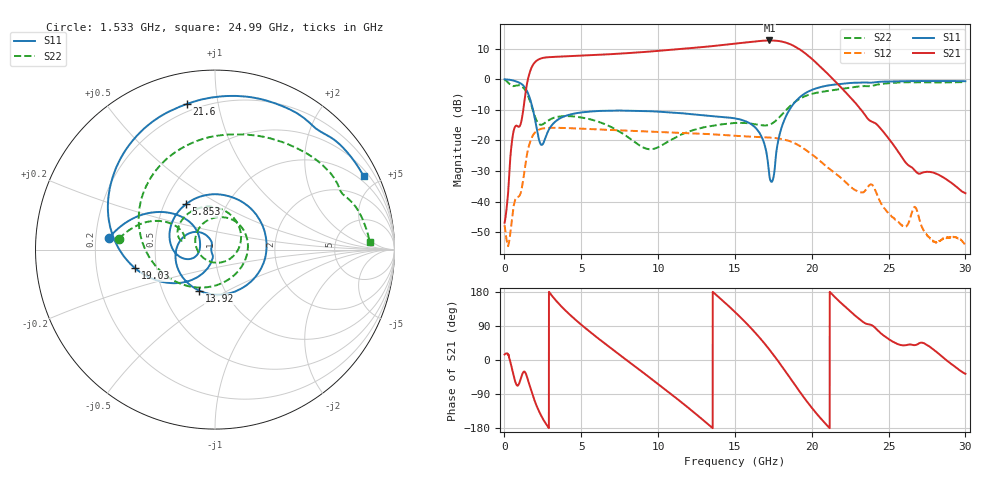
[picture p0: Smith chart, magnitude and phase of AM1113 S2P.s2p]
!Agilent Technologies,E8364B,MY43040894,A.07.50.67
!Agilent E8364B: A.07.50.67
!Date: Thursday, February 22, 2024 05:41:37
!Correction: S11(Full 2 Port(1,2))
!S21(Full 2 Port(1,2))
!S12(Full 2 Port(1,2))
!S22(Full 2 Port(1,2))
!S2P File: Measurements: S11, S21, S12, S22:
# Hz S  dB  R 50
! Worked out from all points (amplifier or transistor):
!   6401 points, 10 MHz to 30 GHz, reference 50 ohm
!   highest |S21| = 12.7 dB at 17.25 GHz (marker M1)
!   |S21| within 3 dB of that: 11.01 GHz to 19.24 GHz (8.229 GHz wide, 54.4 % of centre)
!   unconditionally stable (mu >= 1): 36.32 MHz to end of sweep
!   at 5.005 GHz: K = 1.38, MAG = 8.2 dB, |S12| = -16.2 dB
!   at 15.01 GHz: K = 1.26, MAG = 12.0 dB, |S12| = -18.5 dB
!   at 30 GHz: K = 464.29, MAG = -21.2 dB, |S12| = -54.2 dB
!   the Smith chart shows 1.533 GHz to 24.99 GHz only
!   S11 on the Smith chart (normalised r, x): 1.533 GHz: 0.26, +0.05; 5.853 GHz: 0.64, +0.36; 13.92 GHz: 0.76, -0.37; 19.03 GHz: 0.38, -0.10; 21.6 GHz: 0.16, +0.81; 24.99 GHz: 0.75, +4.19
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1e7  0.01 -7.8  -46.89 14.5  -47.68 160.3  -0.17 -10.7
7.410062e8  -0.65 -89.1  -15.20 -61.4  -38.95 153.5  -2.08 -88.8
1.53293e9  -4.55 173.5  0.14 -53.2  -22.94 141.6  -5.37 173.6
2.043697e9  -14.61 132.1  5.87 -116.0  -17.13 76.4  -12.95 149.9
2.863736e9  -16.72 -159.2  7.23 -178.2  -15.88 11.6  -13.44 161.8
3.913386e9  -12.07 172.8  7.50 132.8  -15.92 -38.3  -12.04 129.1
5.009895e9  -10.83 142.9  7.72 92.7  -16.15 -77.9  -12.48 93.0
5.853364e9  -10.45 122.3  7.92 64.9  -16.33 -104.8  -13.45 65.9
7.999523e9  -10.25 74.0  8.55 -1.8  -16.79 -167.2  -18.77 -12.5
1.000979e10  -10.56 26.0  9.30 -63.7  -17.19 137.1  -22.18 -140.0
1.189354e10  -11.26 -30.5  10.09 -123.8  -17.57 84.7  -17.30 138.7
1.392255e10  -12.22 -110.7  11.06 167.0  -18.08 25.8  -14.86 86.9
1.5005e10  -12.77 -158.7  11.66 126.6  -18.46 -7.4  -14.28 58.3
1.621866e10  -15.27 149.0  12.33 76.6  -18.80 -44.7  -14.59 11.5
1.724956e10  -31.87 139.6  12.70 27.2  -19.03 -80.9  -14.84 -61.3
1.804617e10  -15.62 -120.0  12.34 -16.0  -19.52 -113.8  -11.59 -132.0
1.903022e10  -6.78 -167.0  10.37 -72.9  -21.24 -159.4  -6.96 161.0
2.00049e10  -3.47 151.7  6.70 -126.2  -24.52 157.8  -4.77 115.8
2.159811e10  -1.65 100.8  -1.05 162.3  -31.00 94.9  -3.38 69.3
2.498605e10  -0.69 26.1  -19.22 55.6  -43.69 49.5  -1.28 2.9
2.500479e10  -0.68 25.7  -19.35 55.1  -43.80 48.9  -1.27 2.5
3e10  -0.62 -63.0  -37.24 -36.4  -54.16 -120.0  -0.90 -74.0
